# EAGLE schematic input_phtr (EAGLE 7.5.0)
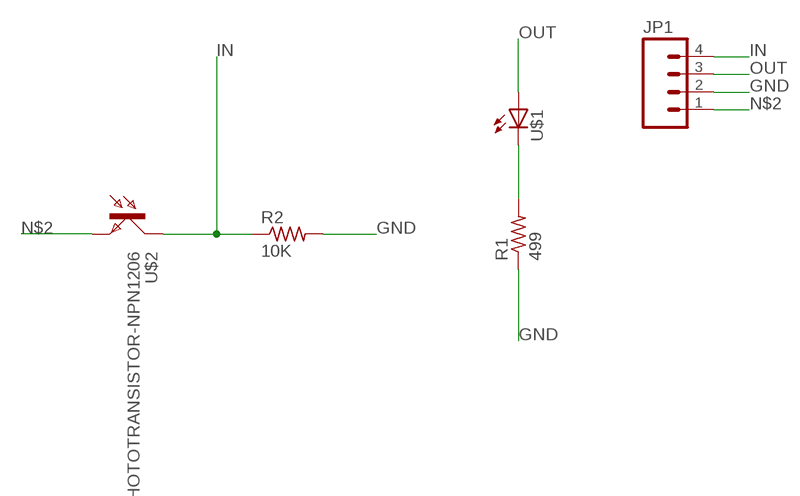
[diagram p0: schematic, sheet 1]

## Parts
JP1  M04SMD  [1X04-SMD]
R1  499  RESISTOR1206  [1206]
R2  10K  RESISTOR1206  [1206]
U$1  LED1206  [1206]
U$2  PHOTOTRANSISTOR-NPN1206  [OP1206]

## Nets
GND: JP1.2 R1.1 R2.2
IN: JP1.4 R2.1 U$2.COLLECTOR(C)
N$1: R1.2 U$1.2(C)
N$2: JP1.1 U$2.EMITTER(E)
OUT: JP1.3 U$1.1(A)

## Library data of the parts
JP1 = 01_SparkFun:M04: Header 4 Standard 4-pin 0.1" header. Use with straight break away headers (SKU : PRT-00116), right angle break away headers (PRT-00553), swiss pins (PRT-00743), machine pins (PRT-00117), and female headers (PRT-00115). Molex polarized connector foot print use with SKU : PRT-08231 with associated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
R1 R2 = 01_FAB_Hello:RESISTOR
U$1 = 01_FAB_Hello:LED
U$2 = 01_fab:PHOTOTRANSISTOR-NPN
